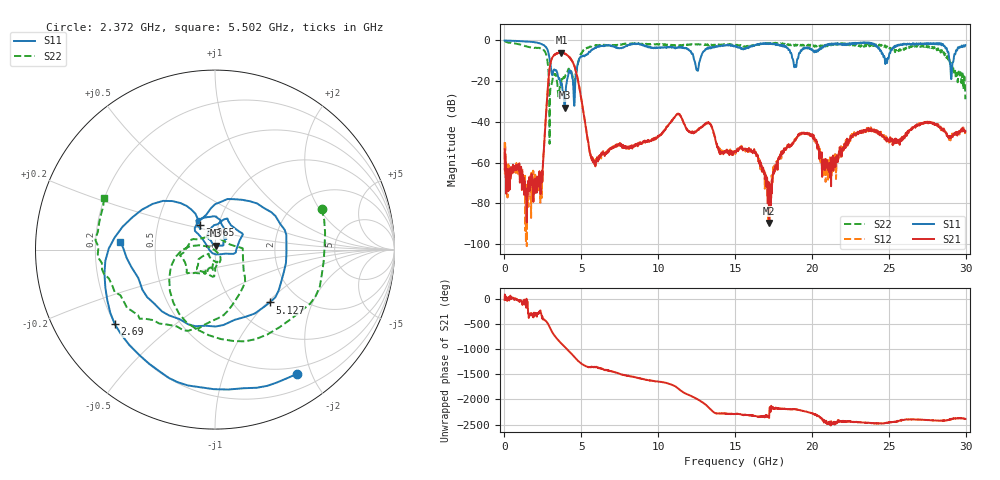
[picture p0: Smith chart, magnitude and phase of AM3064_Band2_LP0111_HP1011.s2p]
# Hz S DB R 50.0
!freq dBS11 angS11 dBS21 angS21 dBS12 angS12 dBS22 angS22
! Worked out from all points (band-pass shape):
!   1600 points, 10 MHz to 29.98 GHz, reference 50 ohm
!   highest |S21| = -5.97 dB at 3.703 GHz (marker M1); lowest = -89.5 dB at 17.22 GHz (marker M2)
!   |S21| within 3 dB of the highest: 3.075 GHz to 4.308 GHz (1.232 GHz wide, 33.4 % of centre)
!   lowest |S11| = -33.0 dB at 3.909 GHz (marker M3), VSWR 1.05, Z = 50.6 + j2.18 ohm
!   |S11| at or under -10 dB: 2.956 GHz to 4.828 GHz (1.871 GHz wide, 48.1 % of centre); 12.36 GHz to 12.71 GHz (346.8 MHz wide, 2.77 % of centre); 28.95 GHz to 29.2 GHz (254.8 MHz wide, 0.876 % of centre)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
!   |S22| runs from -50.7 to -0.2 dB; largest |S21 - S12| = 0.015
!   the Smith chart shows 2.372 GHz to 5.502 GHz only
!   S11 on the Smith chart (normalised r, x): 2.372 GHz: 0.40, -1.78; 2.69 GHz: 0.20, -0.32; 3.065 GHz: 0.81, +0.23; 5.127 GHz: 1.44, -1.04; 5.502 GHz: 0.31, +0.04
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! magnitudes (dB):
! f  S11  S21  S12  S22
! 10 MHz  0.0  -53.4  -49.9  -0.2
! 1.416 GHz  -0.5  -72.9  -77.4  -2.8
! 2.372 GHz  -1.6  -68.0  -73.3  -3.9
! 2.69 GHz  -3.1  -37.5  -37.4  -6.4
! 3.065 GHz  -15.9  -9.2  -9.1  -21.5
! 3.703 GHz  -21.1  -6.0  -6.0  -19.8
! 3.909 GHz  -33.0  -6.5  -6.3  -18.2
! 5.015 GHz  -8.0  -29.4  -29.5  -6.4
! 5.127 GHz  -7.4  -34.8  -34.8  -5.0
! 5.502 GHz  -5.5  -52.9  -52.5  -3.3
! 10 GHz  -3.6  -46.7  -47.1  -2.0
! 11.31 GHz  -3.2  -36.3  -36.0  -2.7
! 15 GHz  -2.7  -54.5  -54.5  -2.0
! 16.34 GHz  -2.4  -54.6  -55.1  -2.5
! 17.22 GHz  -1.4  -89.5  -78.2  -1.5
! 18.25 GHz  -3.3  -53.7  -53.4  -2.0
! 19.99 GHz  -4.4  -46.5  -46.3  -2.2
! 20.93 GHz  -2.2  -62.2  -64.8  -2.3
! 25 GHz  -8.4  -48.8  -48.8  -3.1
! 28.31 GHz  -1.9  -42.7  -42.8  -4.6
! 29.06 GHz  -19.0  -47.7  -48.1  -11.8
! 29.98 GHz  -2.3  -44.6  -44.8  -28.9
